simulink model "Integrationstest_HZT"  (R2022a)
settings: Solver=VariableStepAuto  StartTime=0.0  StopTime=10.0  RelTol=1e-3
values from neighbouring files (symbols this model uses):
  PAR_HZT_MaxLeistung_Heizung = 10000    [parameter_HZT.m]
  PAR_HZT_MaxLeistung_Warmwasser = 4500    [parameter_HZT.m]
  PAR_HZT_MinLeistung_Klima = -10000    [parameter_HZT.m]

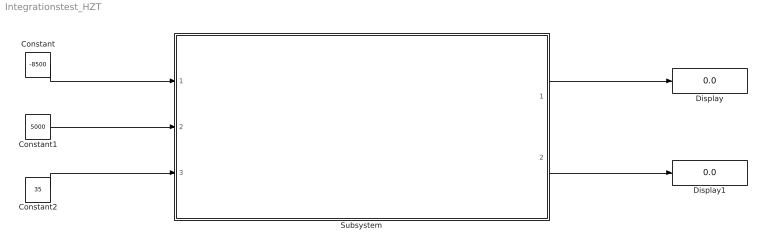
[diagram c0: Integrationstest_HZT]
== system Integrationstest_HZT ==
  Constant : Constant  Value=-8500
  Constant1 : Constant  Value=5000
  Constant2 : Constant  Value=35
  Display : Display
  Display1 : Display
  Subsystem : Subsystem
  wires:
  Subsystem/2(HZT_Warmwasserspeicher_verbrauchte_Leistung) -> Display1/1
  Subsystem/1(HZT_verbrauchte_Leistung) -> Display/1
  Constant2/1 -> Subsystem/3(LKT_Temperatur)
  Constant1/1 -> Subsystem/2(HZR_Warmwasserheizleistung_Waermepumpe)
  Constant/1 -> Subsystem/1(HZR_Heizleistung)

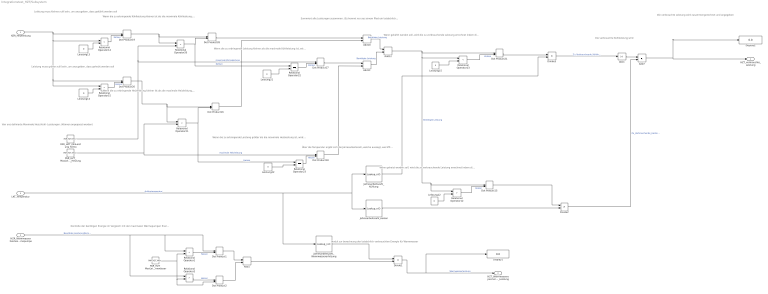
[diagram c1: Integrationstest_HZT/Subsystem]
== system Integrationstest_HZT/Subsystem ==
  note: Kontrolle der benötigen Energie im Vergleich mit der maximalen Wärmepumpen Energie für Warmwasser.
  note: Wenn geheizt werden soll, wird die zu verbrauchende Leistung errechnet indem die Heizleistung durch die Jahresarbeitszahl geteilt wird
  note: Die verbrauchte Leistung wird zusammengerechnet und angegeben
  note: Von uns definierte Maximale Heiz-/kühl- Leistungen. (Können angepasst werden)
  note: Über die Temperatur ergibt sich die Jahresarbeitszahl, welche aussagt, wie Effizient die Wärmepumpe ist.
  note: Modul zur berechnung der tatsächlich verbrauchten Energie für Warmwasser
  note: Wenn die zu erbringende Kühlleistung kleiner ist als die maximale Kühlleistung, kann die angegebene Kühlleistung für die weitere Berechnung genutzt werden.
  note: Wenn die zu erbringende Heizleistung kleiner ist als die maximale Heizleistung, kann die angegebene Heizleistung für die weitere Berechnung genutzt werden.
  note: Die verbrauchte Kühlleistung wird
  note: Leistung muss größer nulll sein, um anzugeben, dass geheizt werden soll
  note: Wenn gekühlt werden soll, wird die zu verbrauchende Leistung errechnet indem die Kühlleistung durch die Jahresarbeitszahl geteilt wird
  note: Wenn die zu erbringende Leistung größer als die maximale Heizleistung ist, wird die maximale Heizleistung angenommen
  note: Summiert alle Leistungen zusammen. (Es kommt nur aus einem Pfad ein tatsächlicher Wert, die anderen ergeben null)
  note: Leistung muss kleiner nulll sein, um anzugeben, dass gekühlt werden soll
  note: Wenn die zu erbringende Leistung kleiner als die maximale Kühlleistung ist, wird die maximale Kühlleistung angenommen
  HZR_Heizleistung : Inport
  HZR_Warmwasserheizleistung_Waermepumpe : Inport  Port=2
  LKT_Temperatur : Inport  Port=3
  Abs1 : Abs
  Add{1,7,10..12} (5 alike) : Sum
  Display1 : Display
  Display2 : Display
  Divide1 : Product  Inputs=/*
  Divide2 : Product  Inputs=*/
  Divide3 : Product  Inputs=*/
  Dot Product{1..2,15..21,28} (10 alike) : DotProduct
  Jahresarbeitszahl_Heizen : Lookup_n-D  NumberOfTableDimensions=1  BreakpointsForDimension1=[-20;-15;-10;-5;0;5;10;20;30]  Table=[1.5;1.7;2.05;2.4;2.7;3;3.2;3.5;3.7]  InternalRulePriority=Speed  RndMeth=Simplest
  Jahresarbeitszahl_Kühlung : Lookup_n-D  NumberOfTableDimensions=1  BreakpointsForDimension1=[20;25;30;35;40]  Table=[3.7;3.2;2.8;2.2;1.5]  InternalRulePriority=Speed  RndMeth=Simplest
  Jahresarbeitszahl_Warmwassererhitzung : Lookup_n-D  NumberOfTableDimensions=1  BreakpointsForDimension1=[-20;-15;-10;-5;0;5;10;15;20;25;30;35;40]  Table=[1.3;1.5;1.7;1.9;2.1;2.3;2.5;2.7;2.9;3.1;3.3;3.5;3.7]  InternalRulePriority=Speed  RndMeth=Simplest
  Leistung{12..15,21..22} (6 alike) : Constant  Value=0
  PAR_HZT_MaxLeistung_Heizung : Constant  Value=PAR_HZT_MaxLeistung_Heizung
  PAR_HZT_MaxLeistung_Warmwasser : Constant  Value=PAR_HZT_MaxLeistung_Warmwasser
  PAR_HZT_MinLeistung_Klima : Constant  Value=PAR_HZT_MinLeistung_Klima
  Relational Operator{1,13..14,21} (4 alike) : RelationalOperator  Operator=<  OutDataTypeStr=boolean  RndMeth=Simplest
  Relational Operator{2,12,15,20} (4 alike) : RelationalOperator  Operator=>  OutDataTypeStr=boolean  RndMeth=Simplest
  Relational Operator22 : RelationalOperator  Operator===  OutDataTypeStr=boolean  RndMeth=Simplest
  Relational Operator23 : RelationalOperator  Operator===  OutDataTypeStr=boolean  RndMeth=Simplest
  HZT_verbrauchte_Leistung : Outport
  HZT_Warmwasserspeicher_verbrauchte_Leistung : Outport  Port=2
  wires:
  PAR_HZT_MinLeistung_Klima/1 -> Dot Product17/1, Relational Operator20/2  "maximale Klimaleistung"
  Dot Product2/1 -> Add1/2
  Relational Operator2/1 -> Dot Product2/1  "Heizen"
  Divide1/1 -> HZT_Warmwasserspeicher_verbrauchte_Leistung/1, Display1/1  "Warmwasserleistung"
  Leistung13/1 -> Relational Operator14/2
  Add7/1 -> HZT_verbrauchte_Leistung/1, Display2/1
  Relational Operator23/1 -> Dot Product18/2  "Heizen"
  Dot Product17/1 -> Add11/1
  Add11/1 -> Add12/2  "Benötigte Leistung"
  Dot Product20/1 -> Dot Product16/1, Relational Operator21/1
  Leistung21/1 -> Relational Operator22/2
  Relational Operator20/1 -> Dot Product28/2, Relational Operator22/1  "Kühlen"
  Leistung12/1 -> Relational Operator12/2
  Relational Operator13/1 -> Dot Product21/2  "Kühlen"
  Add10/1 -> Add12/1  "Benötigte Leistung"
  Leistung22/1 -> Relational Operator23/2
  Add12/1 -> Relational Operator13/1, Relational Operator12/1, Dot Product15/1, Dot Product21/1  "Benötigte Leistung"
  Relational Operator12/1 -> Dot Product15/2  "Heizen"
  Dot Product28/1 -> Add10/1
  Abs1/1 -> Add7/1
  Add1/1 -> Divide1/2
  Dot Product21/1 -> Divide3/1
  Relational Operator15/1 -> Dot Product20/2  "Heizen"
  PAR_HZT_MaxLeistung_Heizung/1 -> Dot Product18/1, Relational Operator21/2  "maximale Heizleistung"
  LKT_Temperatur/1 -> Jahresarbeitszahl_Kühlung/1, Jahresarbeitszahl_Heizen/1, Jahresarbeitszahl_Warmwassererhitzung/1  "Außentemperatur"
  Jahresarbeitszahl_Heizen/1 -> Divide2/2
  Dot Product16/1 -> Add10/2
  PAR_HZT_MaxLeistung_Warmwasser/1 -> Relational Operator2/2, Dot Product2/2, Relational Operator1/2
  Dot Product19/1 -> Dot Product28/1, Relational Operator20/1
  HZR_Heizleistung/1 -> Dot Product19/1, Relational Operator14/1, Dot Product20/1, Relational Operator15/1
  Leistung15/1 -> Relational Operator13/2
  Divide3/1 -> Abs1/1  "Zu_Verbrauchende_Kühlleistung"
  Leistung14/1 -> Relational Operator15/2
  Dot Product18/1 -> Add11/2
  Dot Product15/1 -> Divide2/1
  Jahresarbeitszahl_Warmwassererhitzung/1 -> Divide1/1
  HZR_Warmwasserheizleistung_Waermepumpe/1 -> Relational Operator2/1, Dot Product1/1, Relational Operator1/1  "Benötigte Leistung Warmwasser"
  Dot Product1/1 -> Add1/1
  Divide2/1 -> Add7/2  "Zu_Verbrauchende_Heizleistung"
  Relational Operator22/1 -> Dot Product17/2  "Kühlen"
  Jahresarbeitszahl_Kühlung/1 -> Divide3/2
  Relational Operator14/1 -> Dot Product19/2  "Kühlen"
  Relational Operator1/1 -> Dot Product1/2  "Heizen"
  Relational Operator21/1 -> Relational Operator23/1, Dot Product16/2  "Heizen"
